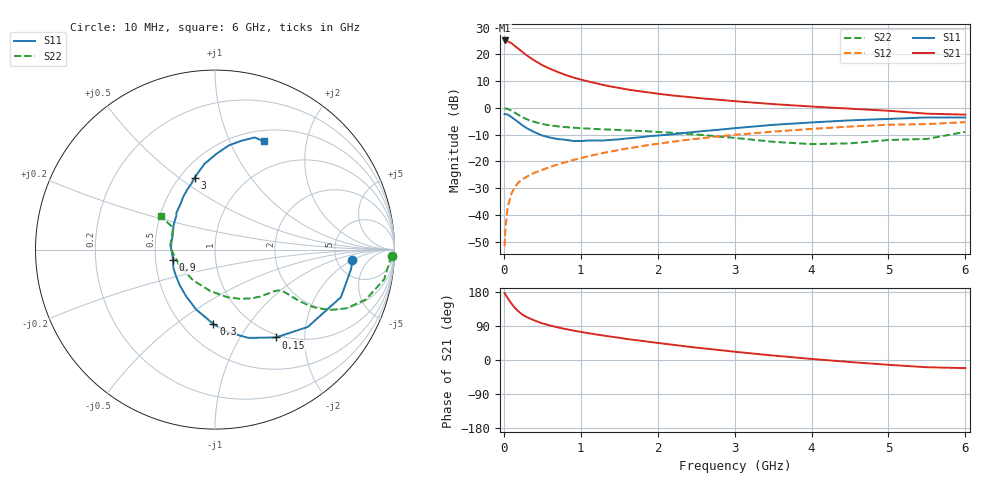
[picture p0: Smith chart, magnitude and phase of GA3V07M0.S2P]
! Infineon Technologies  Discrete & RF Semiconductors
! BF775
! Si NPN RF Bipolar Junction Transistor in SOT23
! VCE = 3 V  IC = 7 mA
! Common Emitter S-Parameters:  May  1996
# GHz  S  MA  R  50
!  f  S11  S21  S12  S22
! GHz  MAG  ANG  MAG  ANG  MAG  ANG  MAG  ANG
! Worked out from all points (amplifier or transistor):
!   36 points, 10 MHz to 6 GHz, reference 50 ohm
!   highest |S21| = 25.2 dB at 10 MHz (marker M1)
!   |S21| within 3 dB of that: start of sweep to 184.9 MHz
!   unconditionally stable (mu >= 1): 673.1 MHz to 3.447 GHz
!   at 250 MHz: K = 0.58, MSG = 23.6 dB, |S12| = -26.6 dB
!   at 1.4 GHz: K = 1.13, MAG = 9.9 dB, |S12| = -16.3 dB
!   at 6 GHz: K = 0.96, MSG = 1.4 dB, |S12| = -5.3 dB
!   S11 on the Smith chart (normalised r, x): 10 MHz: 7.05, -1.98; 150 MHz: 0.95, -1.45; 300 MHz: 0.70, -0.70; 900 MHz: 0.62, -0.08; 3 GHz: 0.59, +0.57; 6 GHz: 0.63, +1.35
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0.01  0.7677 -4.3  18.21 176.6  0.0026 88.1  0.9878 -2.0
0.02  0.7658 -8.2  17.97 172.9  0.0054 85.4  0.9744 -4.1
0.05  0.75 -20.7  17.57 163.3  0.0139 79.3  0.9567 -10.0
0.1  0.673 -39.8  16.11 148.6  0.0254 71.4  0.8855 -18.3
0.15  0.5956 -55.3  14.09 136.0  0.0344 65.3  0.8011 -24.1
0.2  0.5259 -69.3  12.4 126.5  0.0416 62.1  0.7258 -27.6
0.25  0.4632 -81.8  10.84 118.7  0.0469 60.1  0.6601 -29.7
0.3  0.4149 -91.2  9.52 113.0  0.052 59.3  0.6115 -30.8
0.4  0.35 -107.4  7.64 104.2  0.0614 58.3  0.5454 -31.4
0.5  0.3043 -122.5  6.302 96.7  0.0695 58.9  0.4993 -31.4
0.6  0.2785 -135.2  5.38 91.1  0.0785 59.6  0.4711 -31.4
0.7  0.2617 -146.6  4.689 86.1  0.0874 60.4  0.4518 -31.5
0.9  0.2409 -166.0  3.718 77.8  0.106 60.6  0.4267 -32.4
1.1  0.2454 177.7  3.114 70.8  0.1249 60.8  0.4098 -34.2
1.3  0.2463 165.1  2.669 64.4  0.1446 60.1  0.3963 -36.4
1.6  0.2679 149.3  2.218 55.5  0.1738 58.3  0.3788 -40.9
2.2  0.3211 126.4  1.699 40.1  0.2335 53.3  0.3426 -52.5
3  0.4174 105.8  1.335 21.8  0.3135 44.5  0.2751 -75.2
3.5  0.4819 96.9  1.177 11.8  0.3598 38.3  0.2321 -96.5
4.5  0.5846 82.6  0.966 -5.3  0.448 25.1  0.2173 -156.9
5.5  0.6629 70.5  0.779 -19.1  0.4974 10.4  0.2629 152.5
6  0.6611 65.8  0.749 -21.4  0.5418 6.3  0.356 148.2
